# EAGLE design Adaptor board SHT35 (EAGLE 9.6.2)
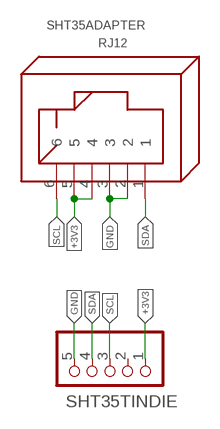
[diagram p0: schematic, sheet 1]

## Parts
SHT35ADAPTER  RJ12  [RJ12]
SHT35TINDIE  PINHD-1X5  [1X05]

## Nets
+3V3: SHT35ADAPTER.4 SHT35ADAPTER.5 SHT35TINDIE.1
GND: SHT35ADAPTER.2 SHT35ADAPTER.3 SHT35TINDIE.5
SCL: SHT35ADAPTER.6 SHT35TINDIE.3
SDA: SHT35ADAPTER.1 SHT35TINDIE.4
Unconnected: SHT35TINDIE.2

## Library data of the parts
SHT35ADAPTER = con-rj:RJ12: RJ12, RJ14 and RJ25 RJ12, RJ14 and RJ25 jacks side mounted http://www.tycoelectronics.com
SHT35TINDIE = pinhead:PINHD-1X5: PIN HEADER

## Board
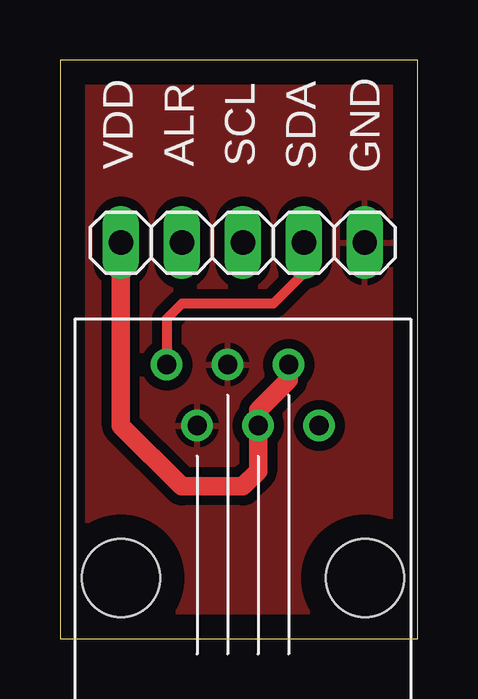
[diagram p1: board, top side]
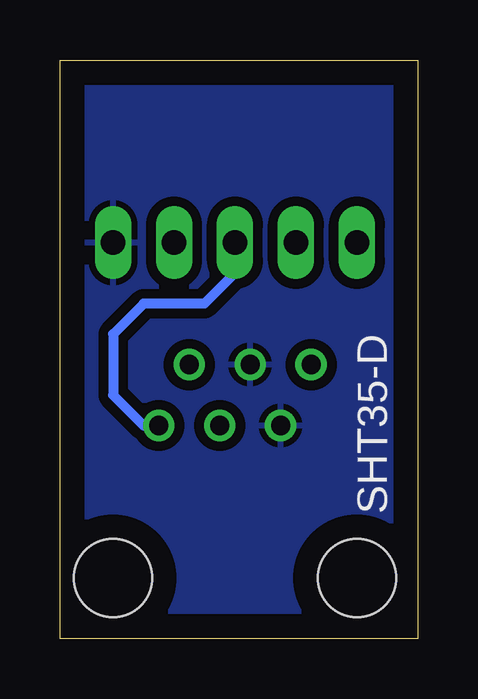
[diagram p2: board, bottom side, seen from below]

Size 14.91 x 24.12 mm. Coordinates in mm from the lower left corner, seen from the top.
Outline: 0,0 14.91,0 14.91,24.12 0,24.12 0,0
Copper layers (1*16): Top 0.035mm / dielectric 1.5mm / Bottom 0.035mm
Design rules "default": minimum track width 6mil, minimum drill 0.35mm, track to track 6mil, track to pad 6mil, pad to pad 6mil, via to via 6mil, smd to smd 6mil, copper to edge 40mil, drill to drill 6mil, minimum pad ring 10mil, minimum via ring 8mil, stop-mask expansion 4mil, vias tented up to drill 0mil, thermal gap 10mil

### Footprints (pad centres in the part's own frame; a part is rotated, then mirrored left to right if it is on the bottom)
RJ12 = drill 0.8: 1 -8.89,-3.175; 2 -6.35,-1.905; 3 -8.89,-0.635; 4 -6.35,0.635; 5 -8.89,1.905; 6 -6.35,3.175 | hole 3.25: 0,-5.08; 0,5.08
1X05 = drill 1.016 long: 1 -5.08,0; 2 -2.54,0; 3 0,0; 4 2.54,0; 5 5.08,0

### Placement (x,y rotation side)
SHT35ADAPTER  7.62,2.54 270 top
SHT35TINDIE  7.62,16.51 0 top

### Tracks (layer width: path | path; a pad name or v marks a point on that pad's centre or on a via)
+3V3
  Top 0.762: SHT35TINDIE.1 2.54,8.89 5.08,6.35 7.62,6.35 8.26,6.98 SHT35ADAPTER.4 8.26,9.52 9.52,10.8 SHT35ADAPTER.5
GND
  pour Bottom (isolate 0.406): 0,24.13 15.24,24.13 15.24,0 0,0
  pour Top (isolate 0.406): 0,24.13 15.24,24.13 15.24,0 0,0
SCL
  Bottom 0.406: SHT35TINDIE.3 7.62,15.24 8.89,13.97 11.43,13.97 12.7,12.7 12.7,10.16 11.43,8.89 SHT35ADAPTER.6
SDA
  Top 0.406: SHT35TINDIE.4 10.16,15.24 8.89,13.97 5.08,13.97 4.45,13.34 SHT35ADAPTER.1

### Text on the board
tPlace: ALR | SCL | VDD | SDA | GND
bPlace: SHT35-D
